| IBIS file stm32u375_385_ufqfpn32.ibs
[IBIS ver] 4.2
[File name] stm32u375_385_ufqfpn32.ibs
[File Rev] 1.2
[Date] 23-06-2025
[Source] Data Created at STMicroelectronics
[Notes]  File originated from ELDO simulations.
[Disclaimer]  This information is for modeling purpose only and is
   not guaranted. The information is subject to change without
   notice.
[Copyright] Copyright 2025 STMicroelectronics Inc.
|   Component stm32u375_385_ufqfpn32
[Component] stm32u375_385_ufqfpn32
[Manufacturer] STMicroelectronics
[Package]
| variable   typ   min   max
R_pkg  0  NA  NA
L_pkg  0  NA  NA
C_pkg  0  NA  NA
[Pin]   signal_name   model_name
0  VSS  gnd
1  VDD  power
2  PC14-OSC32_IN  io_ft_tamp
3  PC15-OSC32_OUT  io_ft_tamp
4  NRST  ioreset_v33
5  VDDA  nc
6  PA0  io8_ft_100m
7  PA1  io8_ft_100m_hslv
8  PA2  io8_ft_100m_hslv
9  PA3  io8_ft_100m_hslv
10  PA4  io8_ft_100m_hslv
11  PA5  io8_ft_100m
12  PA6  io8_ft_100m_hslv
13  PA7  io8_ft_100m_hslv
14  PB0  io8_ft_100m_hslv
15  PB1  io8_ft_100m_hslv
16  VSS  gnd
17  VDD  power
18  PA8  io8_ft_100m_hslv
19  PA9  io8_ft_100m
20  PA10  io8_ft_100m
21  PA11  io8usb_ft_phy
22  PA12  io8usb_ft_phy
23  PA13  io8_ft_100m
24  PA14  io8_ft_100m
25  PA15  io8_ft_100m
26  PB3  io8_ft_100m_hslv
27  PB4  io8_ft_100m_hslv
28  PB5  io8_ft_100m_hslv
29  PB6  io8_ft_100m_hslv
30  PB7  io8_ft_100m_hslv
31  VCAP  nc
32  VSS  gnd
[Package Model]   454-qfpn-5x5-32-ldo-250506
[Pin Mapping]   pulldown_ref   pullup_ref   | Comment
0  gndio  nc
1  nc  vddio
2  gndio  vddio
3  gndio  vddio
4  gndio  vddio
5  nc  nc
6  gndio  vddio
7  gndio  vddio
8  gndio  vddio
9  gndio  vddio
10  gndio  vddio
11  gndio  vddio
12  gndio  vddio
13  gndio  vddio
14  gndio  vddio
15  gndio  vddio
16  gndio  nc
17  nc  vddio
18  gndio  vddio
19  gndio  vddio
20  gndio  vddio
21  gndio  vddio
22  gndio  vddio
23  gndio  vddio
24  gndio  vddio
25  gndio  vddio
26  gndio  vddio
27  gndio  vddio
28  gndio  vddio
29  gndio  vddio
30  gndio  vddio
31  nc  nc
32  gndio  nc
|[Diff Pin]  inv_pin  vdiff  tdelay_typ  tdelay_min  tdelay_max
|22  21  NA  NA  NA  NA
[Model Selector] io8_ft_100m
io8_ft_100m_ls_1v2  "GPIO 100MHz - 5V tolerant - low speed - 1.2V range"
io8_ft_100m_ls_1v8  "GPIO 100MHz - 5V tolerant - low speed - 1.8V range"
io8_ft_100m_ls_3v3  "GPIO 100MHz - 5V tolerant - low speed - 3.3V range"
io8_ft_100m_ms_1v2  "GPIO 100MHz - 5V tolerant - med speed - 1.2V range"
io8_ft_100m_ms_1v8  "GPIO 100MHz - 5V tolerant - med speed - 1.8V range"
io8_ft_100m_ms_3v3  "GPIO 100MHz - 5V tolerant - med speed - 3.3V range"
io8_ft_100m_fs_1v2  "GPIO 100MHz - 5V tolerant - fast speed - 1.2V range"
io8_ft_100m_fs_1v8  "GPIO 100MHz - 5V tolerant - fast speed - 1.8V range"
io8_ft_100m_fs_3v3  "GPIO 100MHz - 5V tolerant - fast speed - 3.3V range"
io8_ft_100m_hs_1v2  "GPIO 100MHz - 5V tolerant - high speed - 1.2V range"
io8_ft_100m_hs_1v8  "GPIO 100MHz - 5V tolerant - high speed - 1.8V range"
io8_ft_100m_hs_3v3  "GPIO 100MHz - 5V tolerant - high speed - 3.3V range"
[Model Selector] io8_ft_100m_hslv
io8_ft_100m_ls_1v2  "GPIO 100MHz - 5V tolerant - low speed - 1.2V range"
io8_ft_100m_ls_1v8  "GPIO 100MHz - 5V tolerant - low speed - 1.8V range"
io8_ft_100m_ls_3v3  "GPIO 100MHz - 5V tolerant - low speed - 3.3V range"
io8_ft_100m_ms_1v2  "GPIO 100MHz - 5V tolerant - med speed - 1.2V range"
io8_ft_100m_ms_1v8  "GPIO 100MHz - 5V tolerant - med speed - 1.8V range"
io8_ft_100m_ms_3v3  "GPIO 100MHz - 5V tolerant - med speed - 3.3V range"
io8_ft_100m_fs_1v2  "GPIO 100MHz - 5V tolerant - fast speed - 1.2V range"
io8_ft_100m_fs_1v8  "GPIO 100MHz - 5V tolerant - fast speed - 1.8V range"
io8_ft_100m_fs_3v3  "GPIO 100MHz - 5V tolerant - fast speed - 3.3V range"
io8_ft_100m_hs_1v2  "GPIO 100MHz - 5V tolerant - high speed - 1.2V range"
io8_ft_100m_hs_1v8  "GPIO 100MHz - 5V tolerant - high speed - 1.8V range"
io8_ft_100m_hs_3v3  "GPIO 100MHz - 5V tolerant - high speed - 3.3V range"
io8_ft_100m_hslv_ls_1v2  "GPIO 100MHz low voltage optimization - 5V tolerant - low speed - 1.2V range"
io8_ft_100m_hslv_ls_1v8  "GPIO 100MHz low voltage optimization - 5V tolerant - low speed - 1.8V range"
io8_ft_100m_hslv_ls_2v5  "GPIO 100MHz low voltage optimization - 5V tolerant - low speed - 3.3V range"
io8_ft_100m_hslv_ms_1v2  "GPIO 100MHz low voltage optimization - 5V tolerant - med speed - 1.2V range"
io8_ft_100m_hslv_ms_1v8  "GPIO 100MHz low voltage optimization - 5V tolerant - med speed - 1.8V range"
io8_ft_100m_hslv_ms_2v5  "GPIO 100MHz low voltage optimization - 5V tolerant - med speed - 3.3V range"
io8_ft_100m_hslv_fs_1v2  "GPIO 100MHz low voltage optimization - 5V tolerant - fast speed - 1.2V range"
io8_ft_100m_hslv_fs_1v8  "GPIO 100MHz low voltage optimization - 5V tolerant - fast speed - 1.8V range"
io8_ft_100m_hslv_fs_2v5  "GPIO 100MHz low voltage optimization - 5V tolerant - fast speed - 3.3V range"
io8_ft_100m_hslv_hs_1v2  "GPIO 100MHz low voltage optimization - 5V tolerant - high speed - 1.2V range"
io8_ft_100m_hslv_hs_1v8  "GPIO 100MHz low voltage optimization - 5V tolerant - high speed - 1.8V range"
io8_ft_100m_hslv_hs_2v5  "GPIO 100MHz low voltage optimization - 5V tolerant - high speed - 3.3V range"
[Model Selector] io8usb_ft_phy
io8_ft_100m_ls_1v2  "GPIO 100MHz - 5V tolerant - low speed - 1.2V range"
io8_ft_100m_ls_1v8  "GPIO 100MHz - 5V tolerant - low speed - 1.8V range"
io8_ft_100m_ls_3v3  "GPIO 100MHz - 5V tolerant - low speed - 3.3V range"
io8_ft_100m_ms_1v2  "GPIO 100MHz - 5V tolerant - med speed - 1.2V range"
io8_ft_100m_ms_1v8  "GPIO 100MHz - 5V tolerant - med speed - 1.8V range"
io8_ft_100m_ms_3v3  "GPIO 100MHz - 5V tolerant - med speed - 3.3V range"
io8_ft_100m_fs_1v2  "GPIO 100MHz - 5V tolerant - fast speed - 1.2V range"
io8_ft_100m_fs_1v8  "GPIO 100MHz - 5V tolerant - fast speed - 1.8V range"
io8_ft_100m_fs_3v3  "GPIO 100MHz - 5V tolerant - fast speed - 3.3V range"
io8_ft_100m_hs_1v2  "GPIO 100MHz - 5V tolerant - high speed - 1.2V range"
io8_ft_100m_hs_1v8  "GPIO 100MHz - 5V tolerant - high speed - 1.8V range"
io8_ft_100m_hs_3v3  "GPIO 100MHz - 5V tolerant - high speed - 3.3V range"
io8usb_ft_phy_hs_3v3   "USB full speed"
io8usb_ft_phy_ls_3v3   "USB low speed"
[Model Selector] io_ft_tamp
io_ft_tamp_ls_1v2 "io8_ft tamp low speed @ 1.2V"
io_ft_tamp_ls_1v8 "io8_ft tamp low speed @ 1.8V"
io_ft_tamp_ls_3v3 "io8_ft tamp low speed @ 3.3V"
io_ft_tamp_ms_1v2 "io8_ft tamp med speed @ 1.2V"
io_ft_tamp_ms_1v8 "io8_ft tamp med speed @ 1.8V"
io_ft_tamp_ms_3v3 "io8_ft tamp med speed @ 3.3V"
io_ft_tamp_fs_1v2 "io8_ft tamp fast speed @ 1.2V"
io_ft_tamp_fs_1v8 "io8_ft tamp fast speed @ 1.8V"
io_ft_tamp_fs_3v3 "io8_ft tamp fast speed @ 3.3V"
io_ft_tamp_hs_1v2 "io8_ft tamp high speed @ 1.2V"
io_ft_tamp_hs_1v8 "io8_ft tamp high speed @ 1.8V"
io_ft_tamp_hs_3v3 "io8_ft tamp high speed @ 3.3V"
[Model Selector] ioreset_v33
ioreset_v33_1v2 "Reset PAD. 5V tolerant. 1.2V range"
ioreset_v33_1v8 "Reset PAD. 5V tolerant. 1.8V range"
ioreset_v33_3v3 "Reset PAD. 5V tolerant. 3.3V range"
[Define Package Model]  454-qfpn-5x5-32-ldo-250506
[Manufacturer]  Unknown
[OEM]  Unknown
[Description]  None
[Number Of Pins]  31
[Pin Numbers]
| Pin Num   Terminal Name
4 | NRST
6 | PA0
7 | PA1
8 | PA2
9 | PA3
10 | PA4
11 | PA5
12 | PA6
13 | PA7
18 | PA8
19 | PA9
20 | PA10
21 | PA11
22 | PA12
23 | PA13
24 | PA14
25 | PA15
14 | PB0
15 | PB1
26 | PB3
27 | PB4
28 | PB5
29 | PB6
30 | PB7
2 | PC14-OSC32_IN
3 | PC15-OSC32_OUT
31 | VCAP
17 | VDD
1 | VDD
5 | VDDA
0 | VSS
|[Merged Pins]  0
|16  |  VSS
|32  |  VSS
[Model Data]
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[End Model Data]
[End Package Model]
|End [Component]
| Models and submodels in the file (41): io8_ft_100m_fs_1v2 (I/O), io8_ft_100m_fs_1v8 (I/O), io8_ft_100m_fs_3v3 (I/O), io8_ft_100m_hs_1v2 (I/O), io8_ft_100m_hs_1v8 (I/O), io8_ft_100m_hs_3v3 (I/O), io8_ft_100m_hslv_fs_1v2 (I/O), io8_ft_100m_hslv_fs_1v8 (I/O), io8_ft_100m_hslv_fs_2v5 (I/O), io8_ft_100m_hslv_hs_1v2 (I/O), io8_ft_100m_hslv_hs_1v8 (I/O), io8_ft_100m_hslv_hs_2v5 (I/O), io8_ft_100m_hslv_ls_1v2 (I/O), io8_ft_100m_hslv_ls_1v8 (I/O), io8_ft_100m_hslv_ls_2v5 (I/O), io8_ft_100m_hslv_ms_1v2 (I/O), io8_ft_100m_hslv_ms_1v8 (I/O), io8_ft_100m_hslv_ms_2v5 (I/O), io8_ft_100m_ls_1v2 (I/O), io8_ft_100m_ls_1v8 (I/O), io8_ft_100m_ls_3v3 (I/O), io8_ft_100m_ms_1v2 (I/O), io8_ft_100m_ms_1v8 (I/O), io8_ft_100m_ms_3v3 (I/O), io8usb_ft_phy_hs_3v3 (I/O), io8usb_ft_phy_ls_3v3 (I/O), io_ft_tamp_fs_1v2 (I/O), io_ft_tamp_fs_1v8 (I/O), io_ft_tamp_fs_3v3 (I/O), io_ft_tamp_hs_1v2 (I/O), io_ft_tamp_hs_1v8 (I/O), io_ft_tamp_hs_3v3 (I/O), io_ft_tamp_ls_1v2 (I/O), io_ft_tamp_ls_1v8 (I/O), io_ft_tamp_ls_3v3 (I/O), io_ft_tamp_ms_1v2 (I/O), io_ft_tamp_ms_1v8 (I/O), io_ft_tamp_ms_3v3 (I/O), ioreset_v33_1v2 (I/O_open_drain), ioreset_v33_1v8 (I/O_open_drain), ioreset_v33_3v3 (I/O_open_drain)
